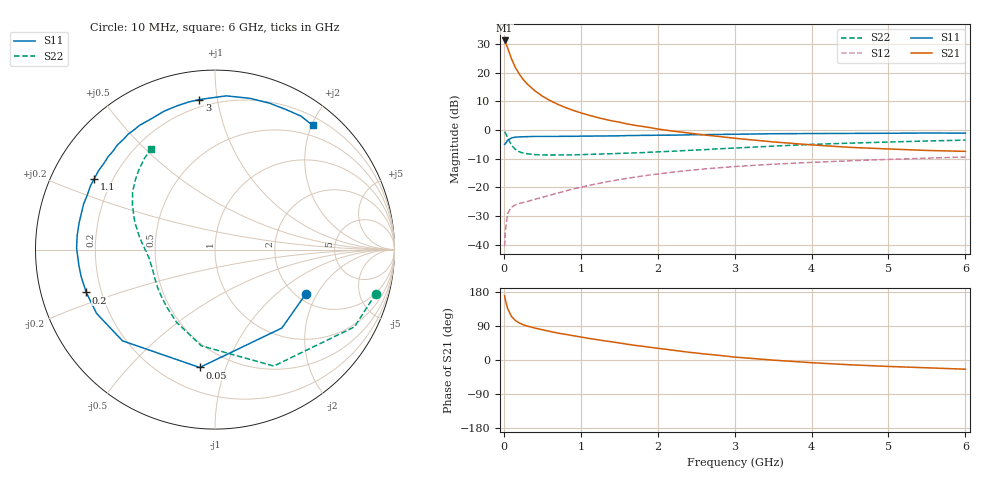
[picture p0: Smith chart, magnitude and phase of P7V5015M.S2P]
! SIEMENS Small Signal Semiconductors
! BFP196
! Si NPN RF Bipolar Junction Transistor in SOT143
! VCE = 0.5 V  IC = 15 mA
! Common Emitter S-Parameters:  May  1996
# GHz  S  MA  R  50
!  f  S11  S21  S12  S22
! GHz  MAG  ANG  MAG  ANG  MAG  ANG  MAG  ANG
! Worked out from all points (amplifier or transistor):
!   36 points, 10 MHz to 6 GHz, reference 50 ohm
!   highest |S21| = 31.2 dB at 10 MHz (marker M1)
!   |S21| within 3 dB of that: start of sweep to 54.58 MHz
!   unconditionally stable (mu >= 1): 668.5 MHz to end of sweep
!   at 250 MHz: K = 0.55, MSG = 21.5 dB, |S12| = -25.3 dB
!   at 1.4 GHz: K = 1.16, MAG = 8.1 dB, |S12| = -17.8 dB
!   at 6 GHz: K = 1.04, MAG = -0.3 dB, |S12| = -9.4 dB
!   S11 on the Smith chart (normalised r, x): 10 MHz: 2.23, -1.62; 50 MHz: 0.35, -0.82; 200 MHz: 0.14, -0.16; 1.1 GHz: 0.13, +0.27; 3 GHz: 0.16, +0.89; 6 GHz: 0.33, +2.02
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0.01  0.5627 -26.2  36.35 169.6  0.0094 79.3  0.9289 -15.3
0.02  0.5743 -49.5  34 158.4  0.0176 71.3  0.8883 -29.0
0.05  0.6623 -97.4  26.79 135.3  0.0351 50.2  0.7269 -63.2
0.1  0.7239 -135.4  17.3 114.6  0.0451 36.1  0.5414 -98.1
0.15  0.7496 -151.7  12.29 104.3  0.0494 31.3  0.458 -117.9
0.2  0.756 -161.6  9.487 97.8  0.0522 30.2  0.4171 -130.4
0.25  0.7607 -168.6  7.624 93.2  0.0542 30.9  0.3951 -139.6
0.3  0.7633 -173.1  6.402 89.8  0.0561 32.3  0.3848 -145.7
0.4  0.7713 179.4  4.857 84.4  0.0617 35.2  0.3719 -154.2
0.5  0.772 174.2  3.894 79.9  0.0668 37.5  0.3664 -159.8
0.6  0.7717 168.8  3.258 75.4  0.0729 40.1  0.3651 -163.8
0.7  0.7716 164.5  2.807 71.1  0.0792 41.9  0.3661 -166.8
0.9  0.7737 157.0  2.197 64.2  0.0933 43.8  0.3676 -171.2
1.1  0.7803 149.5  1.817 57.2  0.1072 44.7  0.3746 -174.6
1.3  0.7834 142.3  1.549 50.9  0.1219 44.3  0.3814 -177.7
1.6  0.7971 133.1  1.274 41.8  0.1431 42.5  0.3946 178.4
2.2  0.8108 115.8  0.953 25.8  0.1839 36.9  0.4257 170.6
3  0.8406 95.9  0.716 7.7  0.2298 26.9  0.4834 158.8
3.5  0.8589 85.8  0.619 -0.3  0.2527 20.7  0.5217 151.8
4.5  0.8706 69.5  0.497 -12.6  0.29 9.4  0.5894 138.9
5.5  0.8848 57.2  0.439 -20.6  0.3224 -1.1  0.6418 127.9
6  0.88 51.8  0.423 -24.3  0.3372 -6.8  0.6649 122.4
